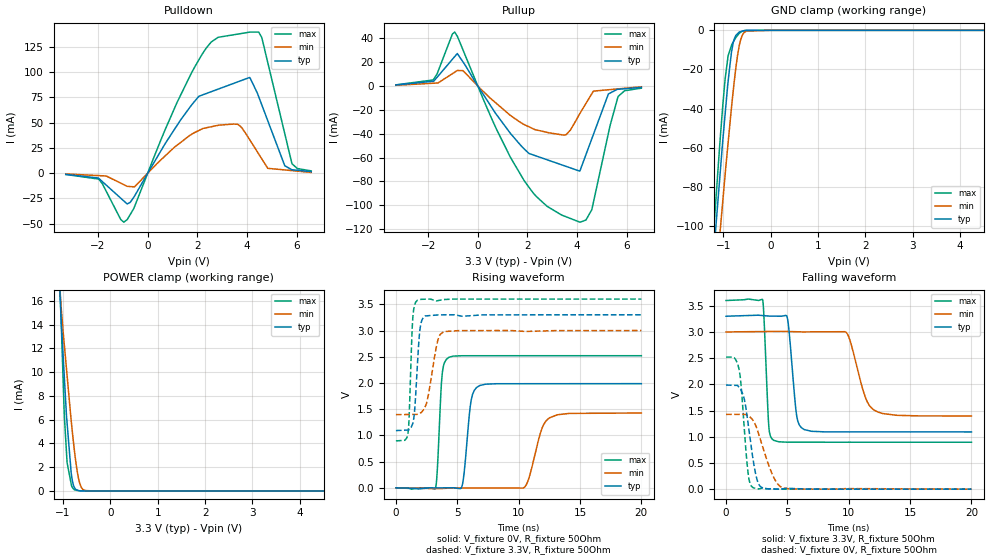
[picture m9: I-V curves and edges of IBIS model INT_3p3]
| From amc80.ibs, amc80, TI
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|   INT model
[Model]  INT_3p3
Model_type   3-state
Polarity   Non-Inverting
Vmeas = 1.65
Vref = 1.65
Cref = 15pF
Rref = 50
|   typ   min   max
|   (nom PVT)   (Fast PVT)   (slow PVT)
|   BUFFER OUTPUT HIGH
|C_comp   1.214E-12   1.214E-12   1.214E-12
|   BUFFER OUTPUT LOW
C_comp   1.459E-12   1.439E-12   1.493E-12
|   BUFFER HIGH Z STATE
|C_comp   1.730E-12   1.419E-12   1.837E-12
| Where   nom PVT is  Nominal Process, 3.3V, 27C
|   Fast PVT is Strong Process, 3.6V, -40C
|   Slow PVT is Weak Process, 3.0V, 125C
|C_comp - from L-C Tank method, L = 1nH, peak frequency
[Voltage Range]   3.3   3   3.6
[Temperature Range]   27   125   -40
[Pullup Reference]   3.3   3   3.6
[Pulldown Reference]   0   0   0
[Power Clamp Reference]   3.3   3   3.6
[GND Clamp Reference]   0   0   0
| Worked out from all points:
|   slope of the pulldown table from 0 to 0.495 V, typ, clamps not added: 24.1 ohm
|   slope of the pullup table from 0 to 0.495 V, typ, clamps not added: 31.2 ohm
|   GND clamp passes 1 mA (typ) near -0.67 V on its own axis
|   POWER clamp passes 1 mA (typ) near -0.81 V on its own axis
|   falling waveform, V_fixture 3.3V, R_fixture 50Ohm: 20-80 % time 487ps typ, 1.12ns min, 293ps max; typ from 3.3 V to 1.09 V
|   rising waveform, V_fixture 0V, R_fixture 50Ohm: 20-80 % time 474ps typ, 957ps min, 305ps max; typ from 0 V to 1.99 V
|   rising waveform, V_fixture 3.3V, R_fixture 50Ohm: 20-80 % time 347ps typ, 692ps min, 241ps max; typ from 1.09 V to 3.3 V
|   falling waveform, V_fixture 0V, R_fixture 50Ohm: 20-80 % time 734ps typ, 1.23ns min, 496ps max; typ from 1.99 V to 0 V
[Pulldown]
|   Voltage   I(typ)   I(min)   I(max)
-3.3V     -1.175mA   -709.3uA   -1.236mA
-1.967V   -5.202mA   -2.389mA   -5.974mA
-958.2mV  -27.52mA   -11.39mA   -48.44mA
-701.6mV  -28.77mA   -13.2mA    -40.79mA
1.313V    52.2mA     30.16mA    76.51mA
2.27V     77.98mA    44.48mA    120.5mA
3.618V    90.24mA    48.46mA    137.6mA
4.126V    94.23mA    32.52mA    139.6mA
4.599V    67.53mA    14.16mA    134.1mA
5.522V    7.519mA    3.246mA    39.33mA
5.811V    3.416mA    2.576mA    9.613mA
6.59V     1.583mA    773.1uA    2.292mA
[GND Clamp]
|   Voltage   I(typ)   I(min)   I(max)
-3.3V     -808.9mA   -769.8mA   -893.6mA
-1.221V   -120.7mA   -146.8mA   -109.1mA
-1.171V   -104.9mA   -132.4mA   -91.86mA
-1.109V   -86.28mA   -114.6mA   -70.64mA
-1.071V   -74.82mA   -104.2mA   -57.59mA
-1.016V   -58.11mA   -89.07mA   -40.26mA
-968.9mV  -45.18mA   -76.17mA   -27.07mA
-897.9mV  -26.2mA    -57.64mA   -13.09mA
-787mV    -6.029mA   -30.41mA   -5.879mA
-662.1mV  -884uA     -7.82mA    -1.506mA
-507.2mV  -49.02uA   -343.9uA   -51.6uA
6.59V     0A         0A         0A
[Pullup]
|   Voltage   I(typ)   I(min)   I(max)
-3.3V     838.5uA    589uA      957.1uA
-1.791V   3.983mA    2.323mA    5.295mA
-930.5mV  24.68mA    11.59mA    45.19mA
-597.2mV  20.18mA    12.87mA    30.22mA
747.1mV   -23.81mA   -14.59mA   -36mA
1.858V    -52.51mA   -32.22mA   -78.97mA
3.545V    -67.31mA   -40.98mA   -109.6mA
4.126V    -70.59mA   -22.57mA   -114.2mA
4.593V    -44.27mA   -6.512mA   -103.7mA
5.259V    -6.793mA   -3.161mA   -39.89mA
5.649V    -2.756mA   -2.426mA   -8.999mA
6.59V     -1.19mA    -650.2uA   -1.826mA
[POWER Clamp]
|   Voltage   I(typ)   I(min)   I(max)
-3.3V     261.6mA    182.4mA    376.9mA
-1.074V   17.54mA    17.25mA    18.57mA
-1.04V    14.51mA    15.55mA    14.52mA
-977.8mV  9.982mA    12.54mA    6.972mA
-926.9mV  6.352mA    10.3mA     3.273mA
-913.7mV  5.712mA    9.724mA    2.377mA
-827.5mV  1.525mA    5.931mA    595.4uA
-757.5mV  267.2uA    3.35mA     87.84uA
-709.6mV  76.81uA    1.892mA    50.37uA
-648.9mV  11.07uA    666.7uA    3.042uA
-529.5mV  419.4nA    32.34uA    2.464uA
6.59V     0A         0A         0A
[Ramp]
R_load = 50
|   typ   min   max
dV/dt_r   1.19193/4.68147e-010  0.856521/9.51951e-010   1.51191/3.04187e-010
dV/dt_f   1.32484/4.84237e-010  0.962182/1.11492e-009   1.62278/2.91304e-010
[Falling Waveform]
V_fixture = 3.3V
V_fixture_min = 3V
V_fixture_max = 3.6V
R_fixture = 50Ohm
C_fixture = 0F
|   Time   V(typ)   V(min)   V(max)
0s        3.3V       3V         3.6V
2.979ns   3.313V     3.008V     3.616V
3.484ns   3.304V     3.009V     1.201V
3.886ns   3.302V     3.01V      931.5mV
4.974ns   3.288V     3.009V     896.8mV
5.754ns   1.403V     3.004V     896mV
6.363ns   1.138V     3.001V     896mV
9.791ns   1.093V     2.992V     895.8mV
12.39ns   1.093V     1.471V     895.7mV
20ns      1.092V     1.396V     895.4mV
[Rising Waveform]
V_fixture = 0V
V_fixture_min = 0V
V_fixture_max = 0V
R_fixture = 50Ohm
C_fixture = 0F
|   Time   V(typ)   V(min)   V(max)
0s        93.71nV    311.9nV    55.56nV
3.219ns   -593.6uV   -14.33mV   -13.78mV
3.764ns   -288.3uV   -12.18mV   2.157V
4.313ns   18.53uV    -6.192mV   2.489V
5.364ns   15.69mV    -927.2uV   2.519V
6.13ns    1.669V     -1.545mV   2.519V
6.819ns   1.95V      -2.102mV   2.519V
10.46ns   1.986V     8.326mV    2.519V
12.54ns   1.986V     1.338V     2.52V
20ns      1.987V     1.428V     2.52V
[Rising Waveform]
V_fixture = 3.3V
V_fixture_min = 3V
V_fixture_max = 3.6V
R_fixture = 50Ohm
C_fixture = 0F
|   Time   V(typ)   V(min)   V(max)
0s        1.092V     1.396V     895.4mV
984.8ps   1.102V     1.398V     1.044V
1.077ns   1.113V     1.399V     1.362V
1.373ns   1.227V     1.399V     3.233V
1.757ns   2.375V     1.404V     3.579V
2.115ns   3.199V     1.452V     3.596V
2.618ns   3.283V     1.739V     3.599V
3.418ns   3.297V     2.815V     3.57V
3.904ns   3.3V       2.979V     3.591V
20ns      3.3V       3V         3.6V
[Falling Waveform]
|Gnd
V_fixture = 0V
V_fixture_min = 0V
V_fixture_max = 0V
R_fixture = 50Ohm
C_fixture = 0F
|   Time   V(typ)   V(min)   V(max)
0s        1.987V     1.428V     2.52V
1.06ns    1.946V     1.427V     2.287V
1.229ns   1.885V     1.427V     1.973V
1.497ns   1.709V     1.426V     1.122V
1.79ns    1.265V     1.406V     319.6mV
2.221ns   541.5mV    1.303V     26.39mV
2.772ns   55.22mV    966.5mV    10.07mV
3.8ns     4.083mV    266.2mV    3.857mV
4.637ns   6.998mV    23.18mV    448.7uV
20ns      93.72nV    311.5nV    55.59nV
